(* Logix 5000 AddOnInstructionDefinition export Banner_K50Z_Param_v4; software revision 33.00; part 2 of 3 *)
(* tags used below, declared in another part *)
   K50Z : Banner_K50Z_v4;
   Port_Data : Banner_IOL_Port_v4;
   Port : DINT;
   Local_Control : DINT;
   Command_Being_Processed : BOOL;
   Update_Archive : BOOL;
   Index_Write_Inprocess : INT;
   Index_Write_Control : INT;
   Inprocess_Index : DINT;
(* Banner_K50Z_Param_v4, continued *)

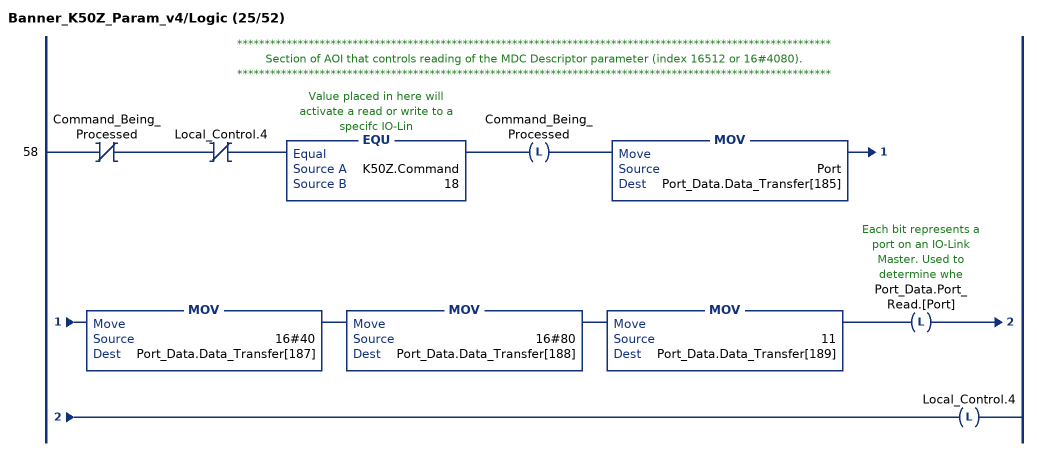
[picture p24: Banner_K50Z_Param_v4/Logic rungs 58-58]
   // ************************************************************************************************************
   // Section of AOI that controls reading of the MDC Descriptor parameter (index 16512 or 16#4080).
   // ************************************************************************************************************
   58: XIO(Command_Being_Processed)XIO(Local_Control.4)EQU(K50Z.Command,18)OTL(Command_Being_Processed)MOV(Port,Port_Data.Data_Transfer[185])MOV(16#40,Port_Data.Data_Transfer[187])MOV(16#80,Port_Data.Data_Transfer[188])MOV(11,Port_Data.Data_Transfer[189])OTL(Port_Data.Port_Read.[Port])OTL(Local_Control.4);
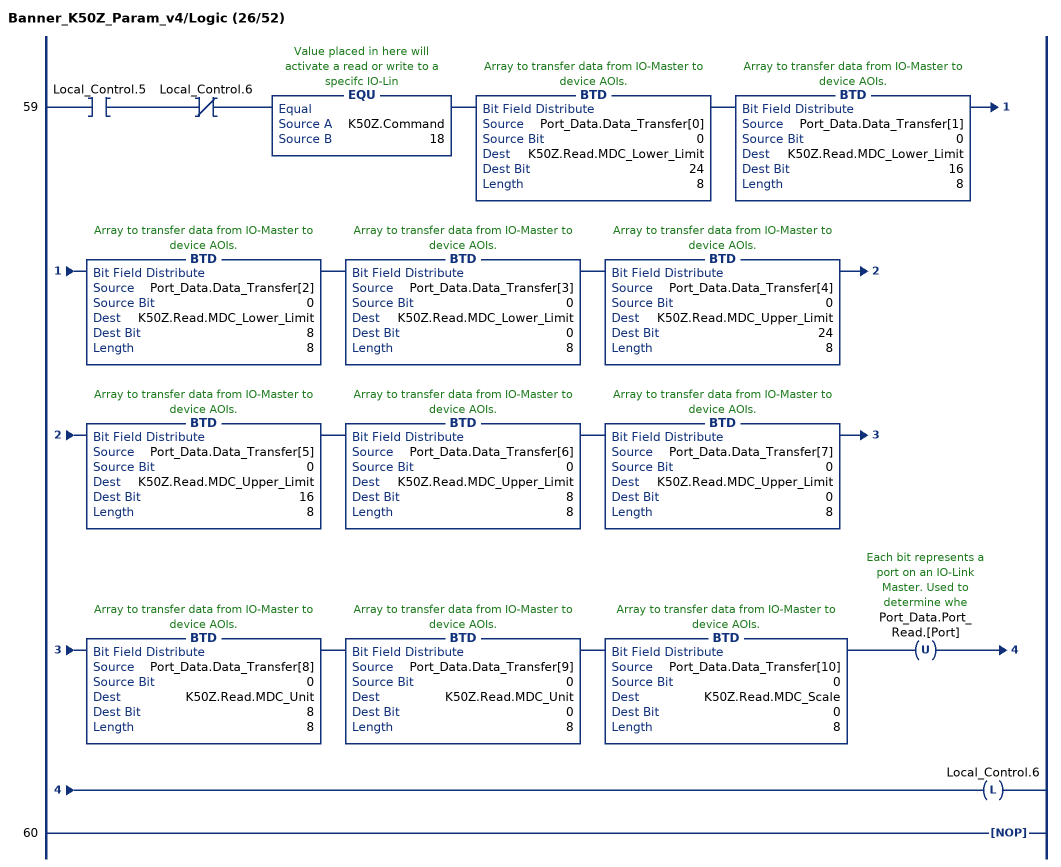
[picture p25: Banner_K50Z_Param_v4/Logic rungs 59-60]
   59: XIC(Local_Control.5)XIO(Local_Control.6)EQU(K50Z.Command,18)BTD(Port_Data.Data_Transfer[0],0,K50Z.Read.MDC_Lower_Limit,24,8)BTD(Port_Data.Data_Transfer[1],0,K50Z.Read.MDC_Lower_Limit,16,8)BTD(Port_Data.Data_Transfer[2],0,K50Z.Read.MDC_Lower_Limit,8,8)BTD(Port_Data.Data_Transfer[3],0,K50Z.Read.MDC_Lower_Limit,0,8)BTD(Port_Data.Data_Transfer[4],0,K50Z.Read.MDC_Upper_Limit,24,8)BTD(Port_Data.Data_Transfer[5],0,K50Z.Read.MDC_Upper_Limit,16,8)BTD(Port_Data.Data_Transfer[6],0,K50Z.Read.MDC_Upper_Limit,8,8)BTD(Port_Data.Data_Transfer[7],0,K50Z.Read.MDC_Upper_Limit,0,8)BTD(Port_Data.Data_Transfer[8],0,K50Z.Read.MDC_Unit,8,8)BTD(Port_Data.Data_Transfer[9],0,K50Z.Read.MDC_Unit,0,8)BTD(Port_Data.Data_Transfer[10],0,K50Z.Read.MDC_Scale,0,8)OTU(Port_Data.Port_Read.[Port])OTL(Local_Control.6);
   60: NOP();
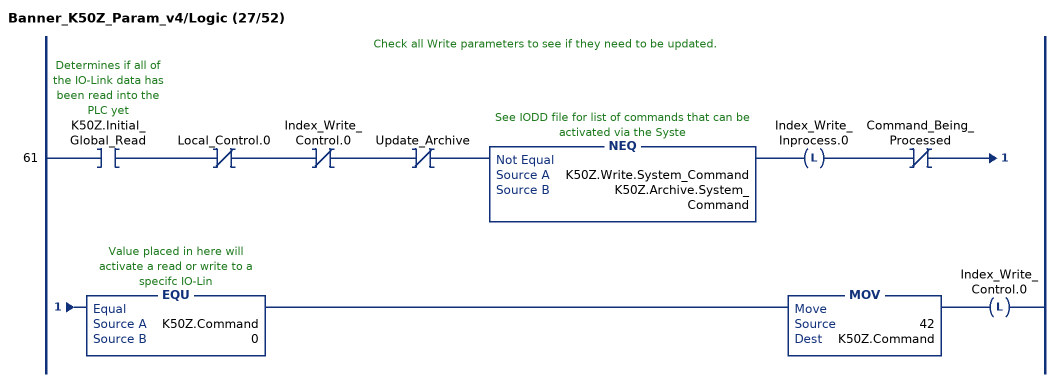
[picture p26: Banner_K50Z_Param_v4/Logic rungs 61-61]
   // Check all Write parameters to see if they need to be updated.
   61: XIC(K50Z.Initial_Global_Read)XIO(Local_Control.0)XIO(Index_Write_Control.0)XIO(Update_Archive)NEQ(K50Z.Write.System_Command,K50Z.Archive.System_Command)OTL(Index_Write_Inprocess.0)XIO(Command_Being_Processed)EQU(K50Z.Command,0)MOV(42,K50Z.Command)OTL(Index_Write_Control.0);
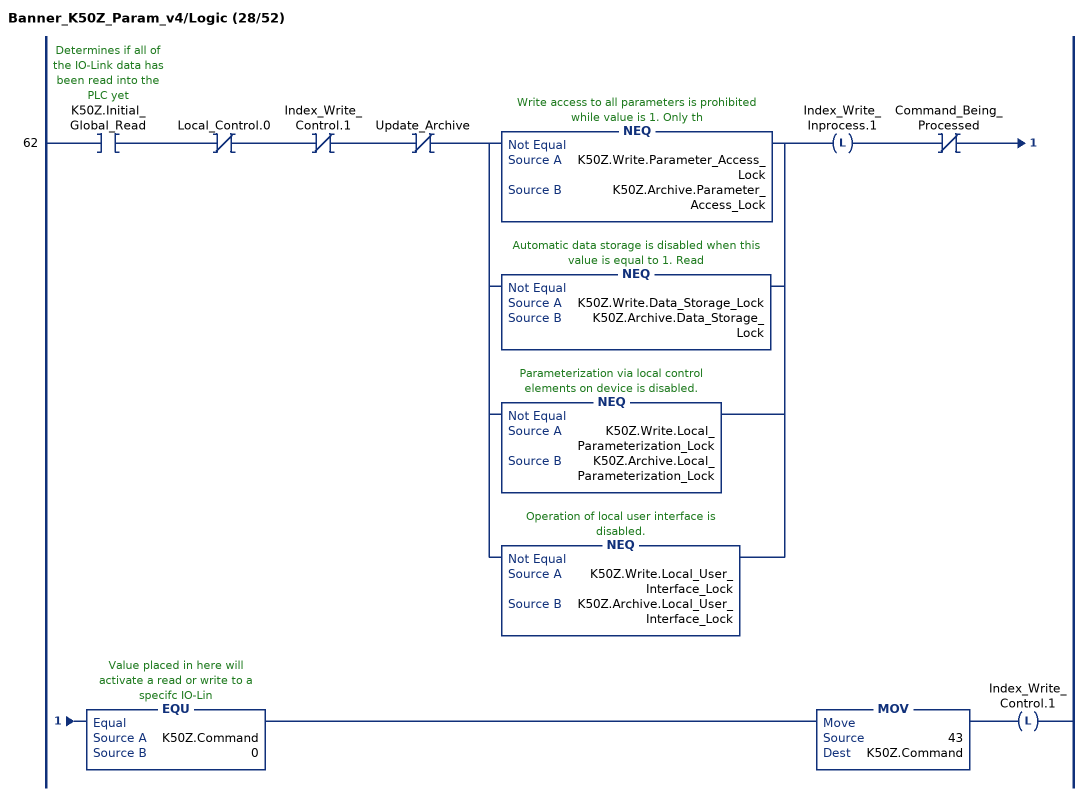
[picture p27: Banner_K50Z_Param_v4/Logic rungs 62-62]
   62: XIC(K50Z.Initial_Global_Read)XIO(Local_Control.0)XIO(Index_Write_Control.1)XIO(Update_Archive)[NEQ(K50Z.Write.Parameter_Access_Lock,K50Z.Archive.Parameter_Access_Lock) ,NEQ(K50Z.Write.Data_Storage_Lock,K50Z.Archive.Data_Storage_Lock) ,NEQ(K50Z.Write.Local_Parameterization_Lock,K50Z.Archive.Local_Parameterization_Lock) ,NEQ(K50Z.Write.Local_User_Interface_Lock,K50Z.Archive.Local_User_Interface_Lock) ]OTL(Index_Write_Inprocess.1)XIO(Command_Being_Processed)EQU(K50Z.Command,0)MOV(43,K50Z.Command)OTL(Index_Write_Control.1);
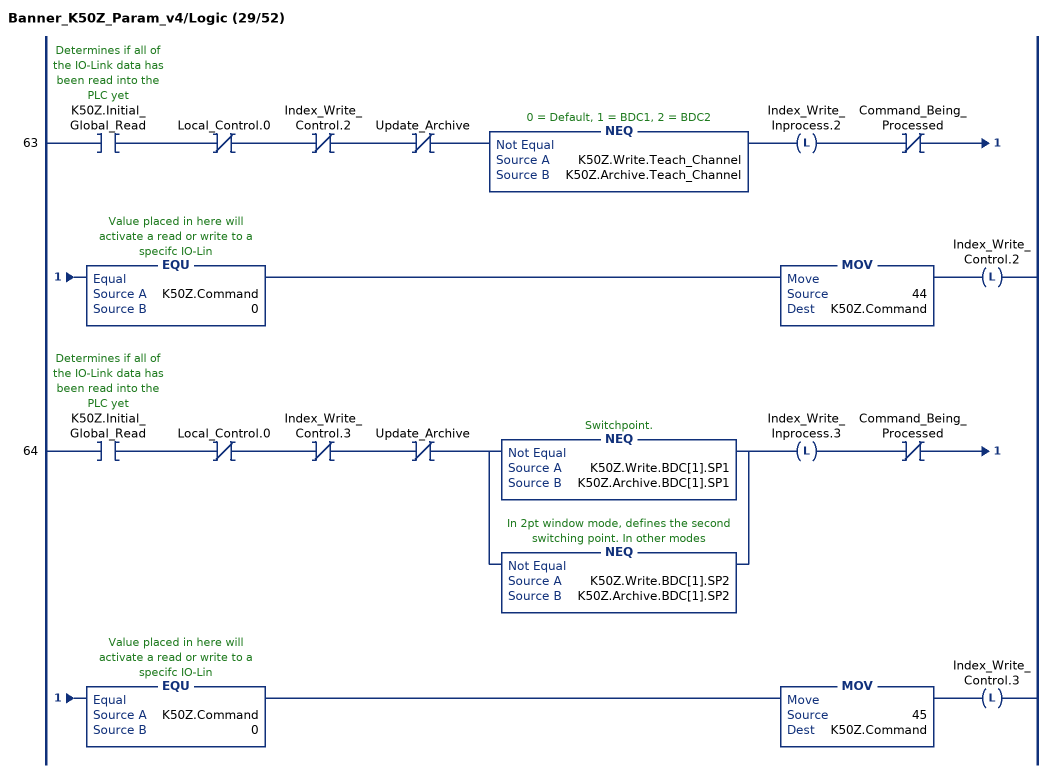
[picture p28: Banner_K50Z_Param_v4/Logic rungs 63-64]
   63: XIC(K50Z.Initial_Global_Read)XIO(Local_Control.0)XIO(Index_Write_Control.2)XIO(Update_Archive)NEQ(K50Z.Write.Teach_Channel,K50Z.Archive.Teach_Channel)OTL(Index_Write_Inprocess.2)XIO(Command_Being_Processed)EQU(K50Z.Command,0)MOV(44,K50Z.Command)OTL(Index_Write_Control.2);
   64: XIC(K50Z.Initial_Global_Read)XIO(Local_Control.0)XIO(Index_Write_Control.3)XIO(Update_Archive)[NEQ(K50Z.Write.BDC[1].SP1,K50Z.Archive.BDC[1].SP1) ,NEQ(K50Z.Write.BDC[1].SP2,K50Z.Archive.BDC[1].SP2) ]OTL(Index_Write_Inprocess.3)XIO(Command_Being_Processed)EQU(K50Z.Command,0)MOV(45,K50Z.Command)OTL(Index_Write_Control.3);
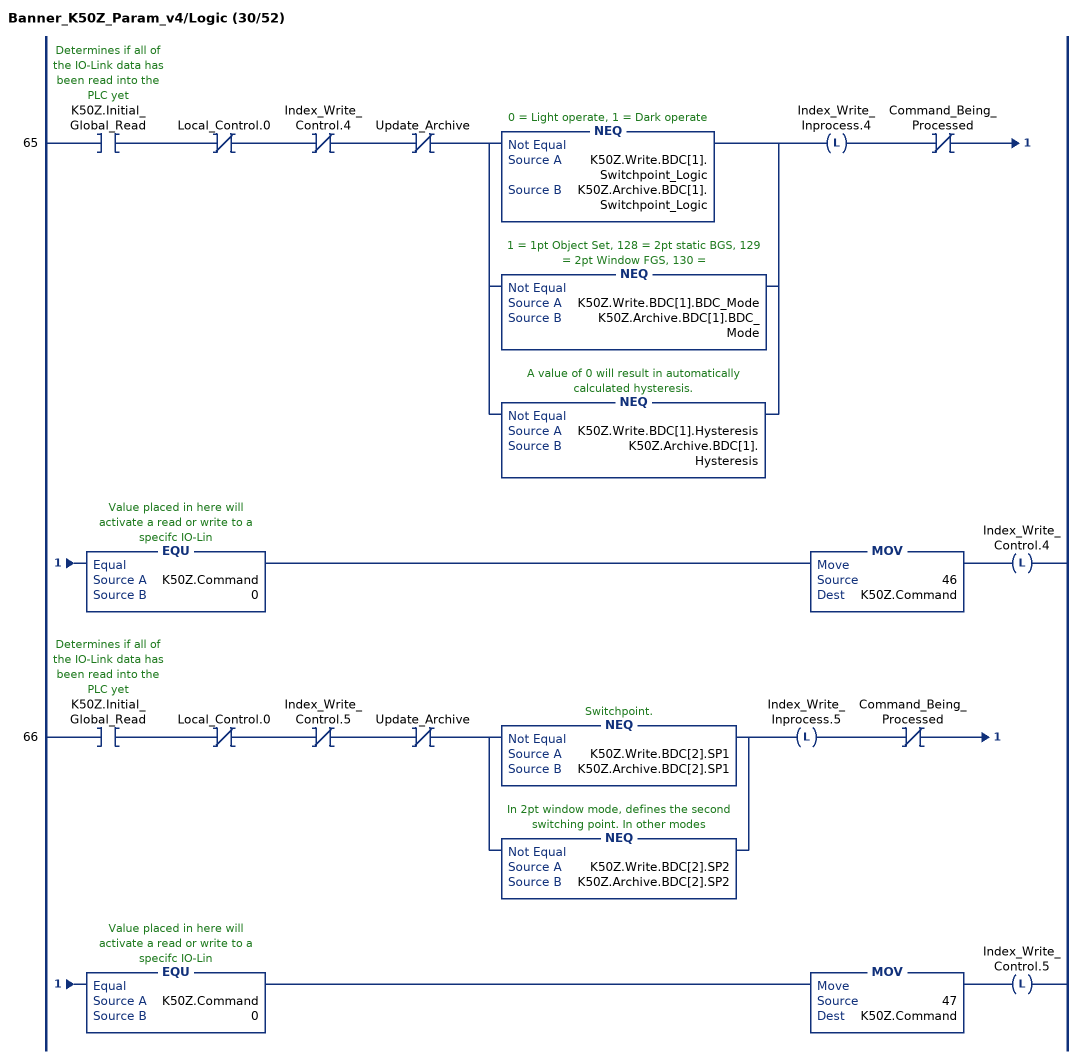
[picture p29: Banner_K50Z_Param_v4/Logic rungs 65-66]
   65: XIC(K50Z.Initial_Global_Read)XIO(Local_Control.0)XIO(Index_Write_Control.4)XIO(Update_Archive)[NEQ(K50Z.Write.BDC[1].Switchpoint_Logic,K50Z.Archive.BDC[1].Switchpoint_Logic) ,NEQ(K50Z.Write.BDC[1].BDC_Mode,K50Z.Archive.BDC[1].BDC_Mode) ,NEQ(K50Z.Write.BDC[1].Hysteresis,K50Z.Archive.BDC[1].Hysteresis) ]OTL(Index_Write_Inprocess.4)XIO(Command_Being_Processed)EQU(K50Z.Command,0)MOV(46,K50Z.Command)OTL(Index_Write_Control.4);
   66: XIC(K50Z.Initial_Global_Read)XIO(Local_Control.0)XIO(Index_Write_Control.5)XIO(Update_Archive)[NEQ(K50Z.Write.BDC[2].SP1,K50Z.Archive.BDC[2].SP1) ,NEQ(K50Z.Write.BDC[2].SP2,K50Z.Archive.BDC[2].SP2) ]OTL(Index_Write_Inprocess.5)XIO(Command_Being_Processed)EQU(K50Z.Command,0)MOV(47,K50Z.Command)OTL(Index_Write_Control.5);
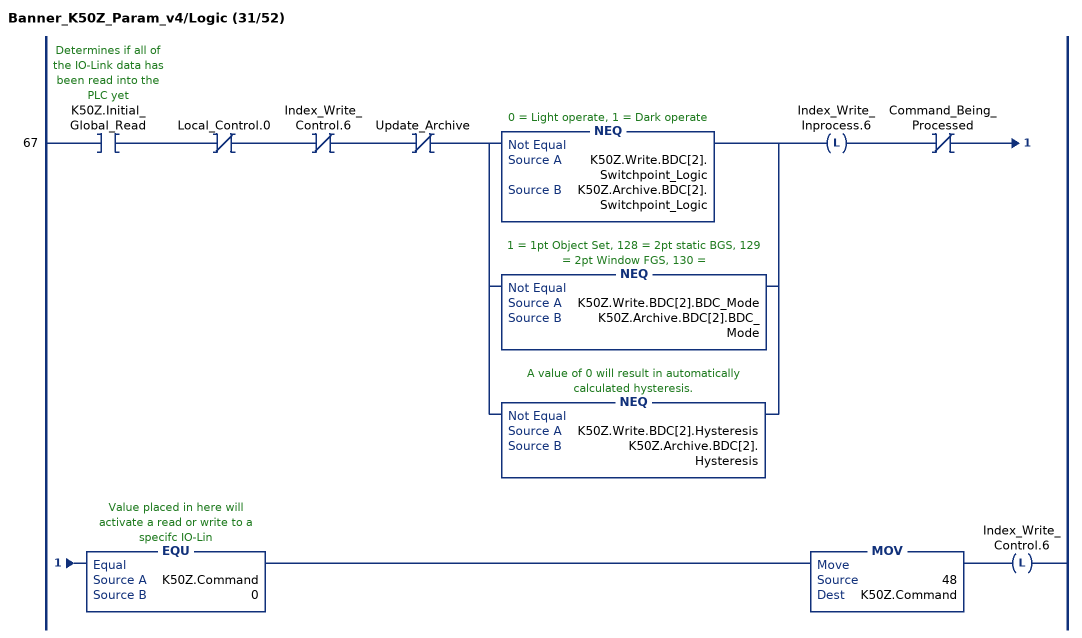
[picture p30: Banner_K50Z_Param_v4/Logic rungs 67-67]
   67: XIC(K50Z.Initial_Global_Read)XIO(Local_Control.0)XIO(Index_Write_Control.6)XIO(Update_Archive)[NEQ(K50Z.Write.BDC[2].Switchpoint_Logic,K50Z.Archive.BDC[2].Switchpoint_Logic) ,NEQ(K50Z.Write.BDC[2].BDC_Mode,K50Z.Archive.BDC[2].BDC_Mode) ,NEQ(K50Z.Write.BDC[2].Hysteresis,K50Z.Archive.BDC[2].Hysteresis) ]OTL(Index_Write_Inprocess.6)XIO(Command_Being_Processed)EQU(K50Z.Command,0)MOV(48,K50Z.Command)OTL(Index_Write_Control.6);
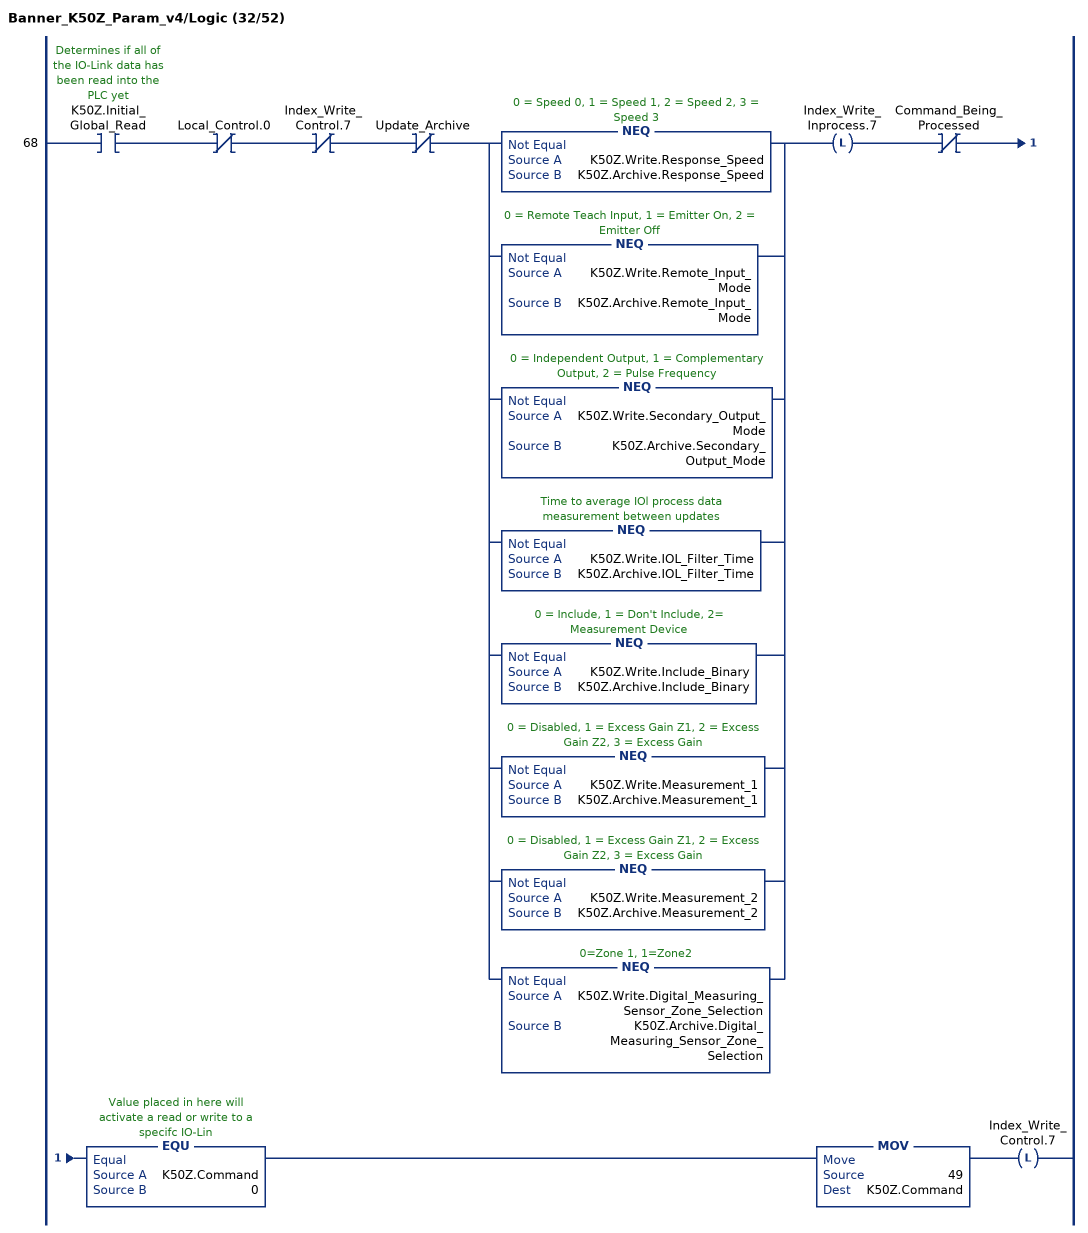
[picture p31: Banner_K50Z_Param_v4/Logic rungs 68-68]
   68: XIC(K50Z.Initial_Global_Read)XIO(Local_Control.0)XIO(Index_Write_Control.7)XIO(Update_Archive)[NEQ(K50Z.Write.Response_Speed,K50Z.Archive.Response_Speed) ,NEQ(K50Z.Write.Remote_Input_Mode,K50Z.Archive.Remote_Input_Mode) ,NEQ(K50Z.Write.Secondary_Output_Mode,K50Z.Archive.Secondary_Output_Mode) ,NEQ(K50Z.Write.IOL_Filter_Time,K50Z.Archive.IOL_Filter_Time) ,NEQ(K50Z.Write.Include_Binary,K50Z.Archive.Include_Binary) ,NEQ(K50Z.Write.Measurement_1,K50Z.Archive.Measurement_1) ,NEQ(K50Z.Write.Measurement_2,K50Z.Archive.Measurement_2) ,NEQ(K50Z.Write.Digital_Measuring_Sensor_Zone_Selection,K50Z.Archive.Digital_Measuring_Sensor_Zone_Selection) ]OTL(Index_Write_Inprocess.7)XIO(Command_Being_Processed)EQU(K50Z.Command,0)MOV(49,K50Z.Command)OTL(Index_Write_Control.7);
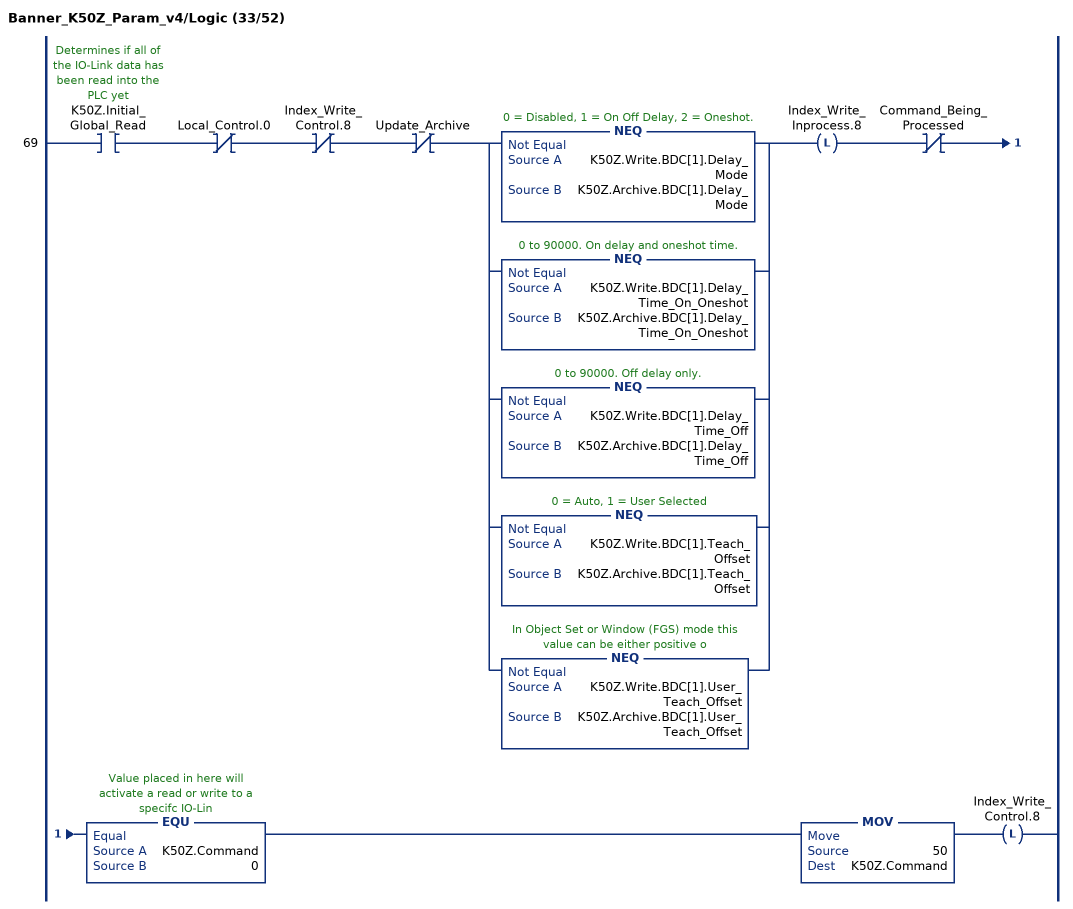
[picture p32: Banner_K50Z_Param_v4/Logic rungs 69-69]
   69: XIC(K50Z.Initial_Global_Read)XIO(Local_Control.0)XIO(Index_Write_Control.8)XIO(Update_Archive)[NEQ(K50Z.Write.BDC[1].Delay_Mode,K50Z.Archive.BDC[1].Delay_Mode) ,NEQ(K50Z.Write.BDC[1].Delay_Time_On_Oneshot,K50Z.Archive.BDC[1].Delay_Time_On_Oneshot) ,NEQ(K50Z.Write.BDC[1].Delay_Time_Off,K50Z.Archive.BDC[1].Delay_Time_Off) ,NEQ(K50Z.Write.BDC[1].Teach_Offset,K50Z.Archive.BDC[1].Teach_Offset) ,NEQ(K50Z.Write.BDC[1].User_Teach_Offset,K50Z.Archive.BDC[1].User_Teach_Offset) ]OTL(Index_Write_Inprocess.8)XIO(Command_Being_Processed)EQU(K50Z.Command,0)MOV(50,K50Z.Command)OTL(Index_Write_Control.8);
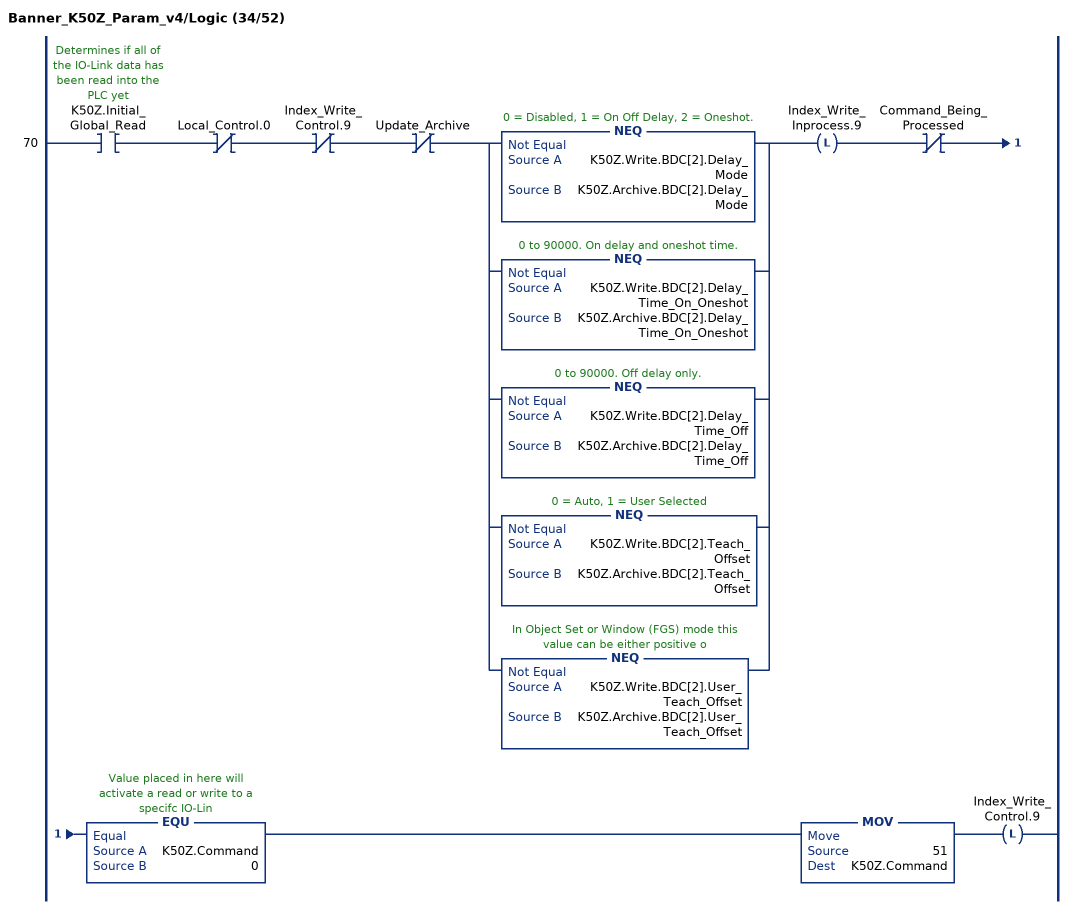
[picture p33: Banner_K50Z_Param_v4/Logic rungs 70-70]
   70: XIC(K50Z.Initial_Global_Read)XIO(Local_Control.0)XIO(Index_Write_Control.9)XIO(Update_Archive)[NEQ(K50Z.Write.BDC[2].Delay_Mode,K50Z.Archive.BDC[2].Delay_Mode) ,NEQ(K50Z.Write.BDC[2].Delay_Time_On_Oneshot,K50Z.Archive.BDC[2].Delay_Time_On_Oneshot) ,NEQ(K50Z.Write.BDC[2].Delay_Time_Off,K50Z.Archive.BDC[2].Delay_Time_Off) ,NEQ(K50Z.Write.BDC[2].Teach_Offset,K50Z.Archive.BDC[2].Teach_Offset) ,NEQ(K50Z.Write.BDC[2].User_Teach_Offset,K50Z.Archive.BDC[2].User_Teach_Offset) ]OTL(Index_Write_Inprocess.9)XIO(Command_Being_Processed)EQU(K50Z.Command,0)MOV(51,K50Z.Command)OTL(Index_Write_Control.9);
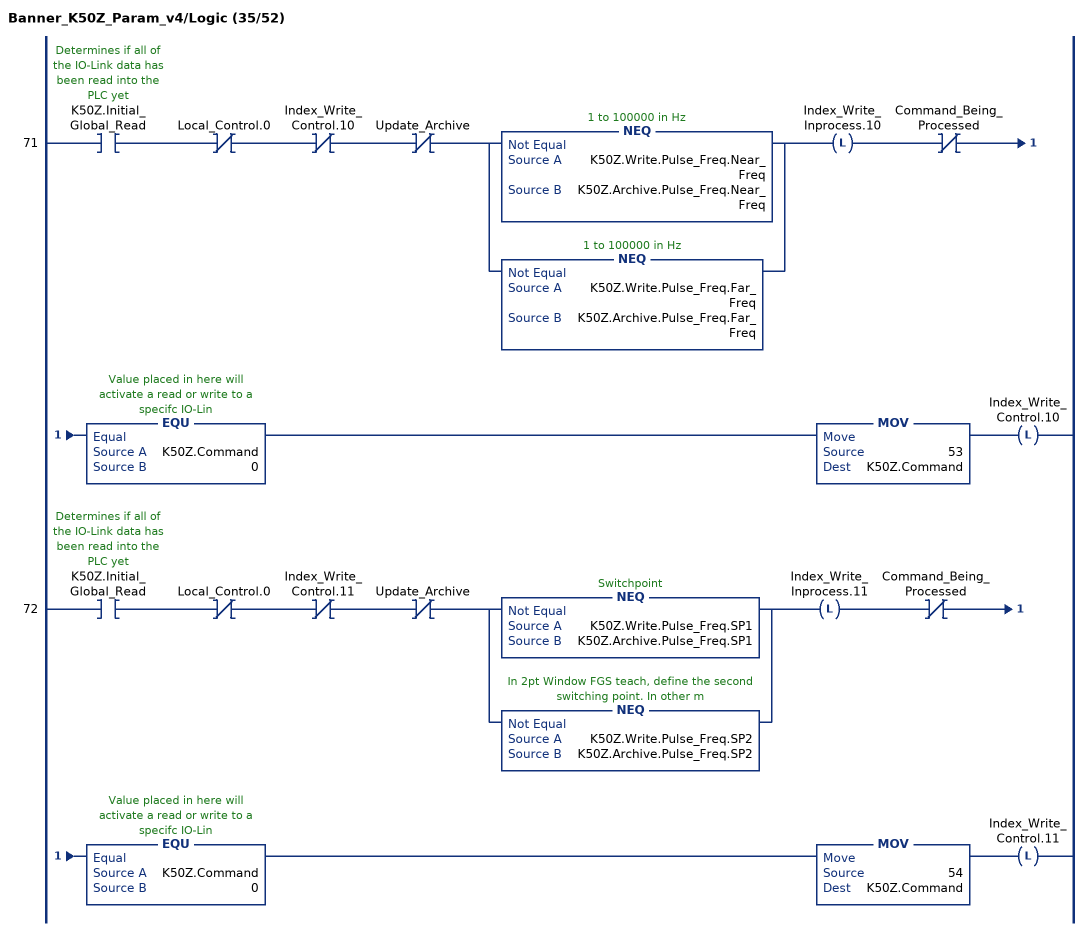
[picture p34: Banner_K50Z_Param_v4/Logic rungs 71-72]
   71: XIC(K50Z.Initial_Global_Read)XIO(Local_Control.0)XIO(Index_Write_Control.10)XIO(Update_Archive)[NEQ(K50Z.Write.Pulse_Freq.Near_Freq,K50Z.Archive.Pulse_Freq.Near_Freq) ,NEQ(K50Z.Write.Pulse_Freq.Far_Freq,K50Z.Archive.Pulse_Freq.Far_Freq) ]OTL(Index_Write_Inprocess.10)XIO(Command_Being_Processed)EQU(K50Z.Command,0)MOV(53,K50Z.Command)OTL(Index_Write_Control.10);
   72: XIC(K50Z.Initial_Global_Read)XIO(Local_Control.0)XIO(Index_Write_Control.11)XIO(Update_Archive)[NEQ(K50Z.Write.Pulse_Freq.SP1,K50Z.Archive.Pulse_Freq.SP1) ,NEQ(K50Z.Write.Pulse_Freq.SP2,K50Z.Archive.Pulse_Freq.SP2) ]OTL(Index_Write_Inprocess.11)XIO(Command_Being_Processed)EQU(K50Z.Command,0)MOV(54,K50Z.Command)OTL(Index_Write_Control.11);
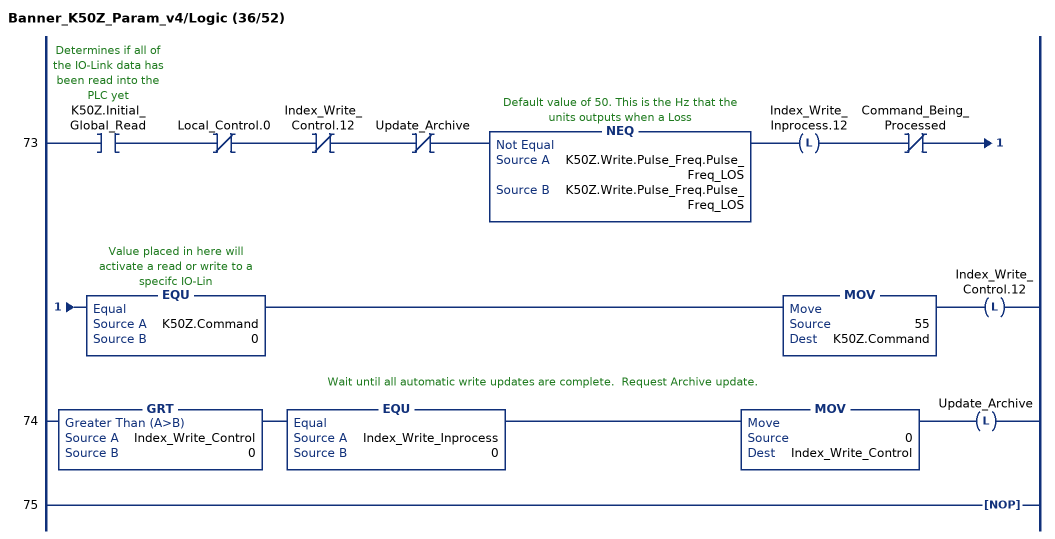
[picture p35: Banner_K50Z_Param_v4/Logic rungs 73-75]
   73: XIC(K50Z.Initial_Global_Read)XIO(Local_Control.0)XIO(Index_Write_Control.12)XIO(Update_Archive)NEQ(K50Z.Write.Pulse_Freq.Pulse_Freq_LOS,K50Z.Write.Pulse_Freq.Pulse_Freq_LOS)OTL(Index_Write_Inprocess.12)XIO(Command_Being_Processed)EQU(K50Z.Command,0)MOV(55,K50Z.Command)OTL(Index_Write_Control.12);
   // Wait until all automatic write updates are complete.  Request Archive update.
   74: GRT(Index_Write_Control,0)EQU(Index_Write_Inprocess,0)MOV(0,Index_Write_Control)OTL(Update_Archive);
   75: NOP();
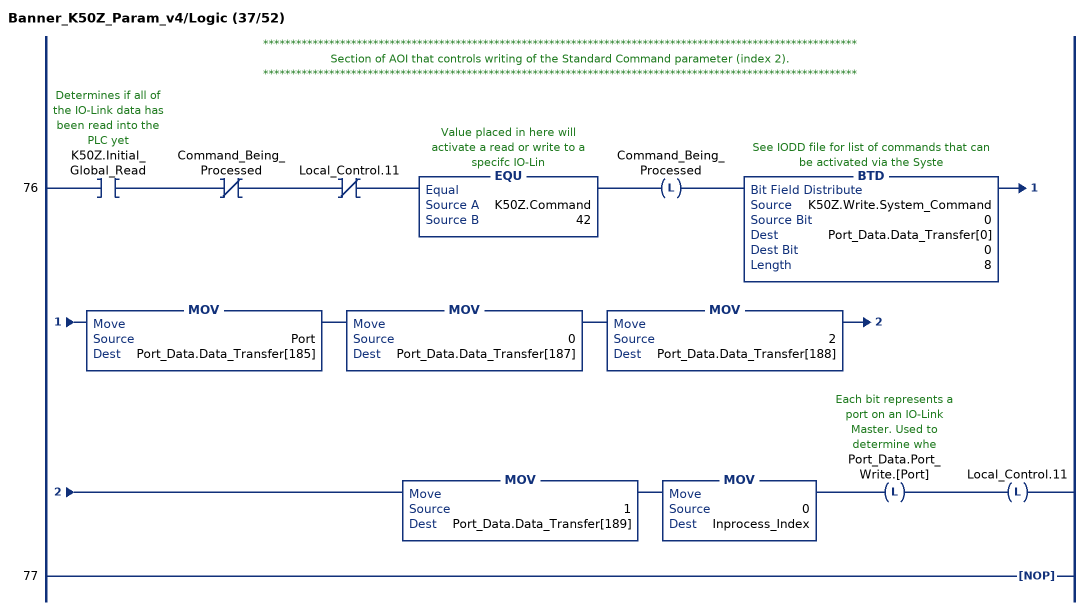
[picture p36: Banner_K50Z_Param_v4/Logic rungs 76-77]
   // ************************************************************************************************************
   // Section of AOI that controls writing of the Standard Command parameter (index 2).
   // ************************************************************************************************************
   76: XIC(K50Z.Initial_Global_Read)XIO(Command_Being_Processed)XIO(Local_Control.11)EQU(K50Z.Command,42)OTL(Command_Being_Processed)BTD(K50Z.Write.System_Command,0,Port_Data.Data_Transfer[0],0,8)MOV(Port,Port_Data.Data_Transfer[185])MOV(0,Port_Data.Data_Transfer[187])MOV(2,Port_Data.Data_Transfer[188])MOV(1,Port_Data.Data_Transfer[189])MOV(0,Inprocess_Index)OTL(Port_Data.Port_Write.[Port])OTL(Local_Control.11);
   77: NOP();
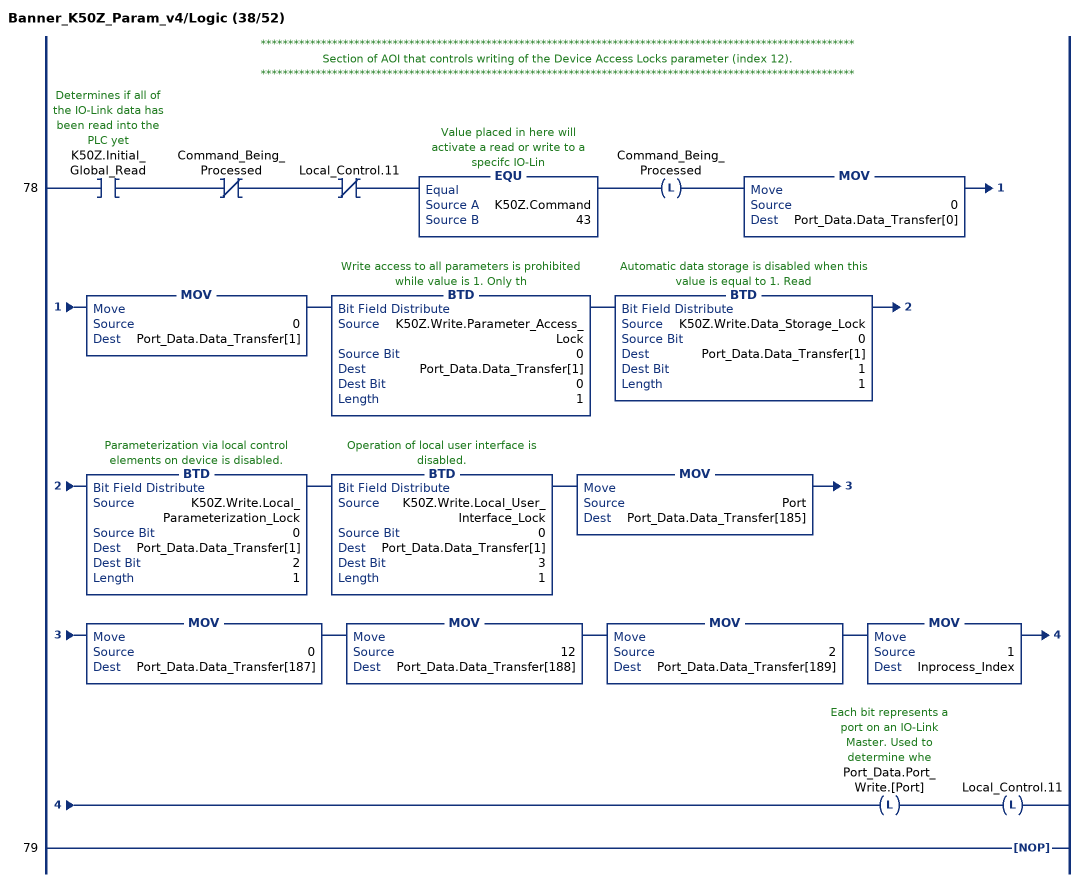
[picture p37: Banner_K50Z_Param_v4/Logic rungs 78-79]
   // ************************************************************************************************************
   // Section of AOI that controls writing of the Device Access Locks parameter (index 12).
   // ************************************************************************************************************
   78: XIC(K50Z.Initial_Global_Read)XIO(Command_Being_Processed)XIO(Local_Control.11)EQU(K50Z.Command,43)OTL(Command_Being_Processed)MOV(0,Port_Data.Data_Transfer[0])MOV(0,Port_Data.Data_Transfer[1])BTD(K50Z.Write.Parameter_Access_Lock,0,Port_Data.Data_Transfer[1],0,1)BTD(K50Z.Write.Data_Storage_Lock,0,Port_Data.Data_Transfer[1],1,1)BTD(K50Z.Write.Local_Parameterization_Lock,0,Port_Data.Data_Transfer[1],2,1)BTD(K50Z.Write.Local_User_Interface_Lock,0,Port_Data.Data_Transfer[1],3,1)MOV(Port,Port_Data.Data_Transfer[185])MOV(0,Port_Data.Data_Transfer[187])MOV(12,Port_Data.Data_Transfer[188])MOV(2,Port_Data.Data_Transfer[189])MOV(1,Inprocess_Index)OTL(Port_Data.Port_Write.[Port])OTL(Local_Control.11);
   79: NOP();
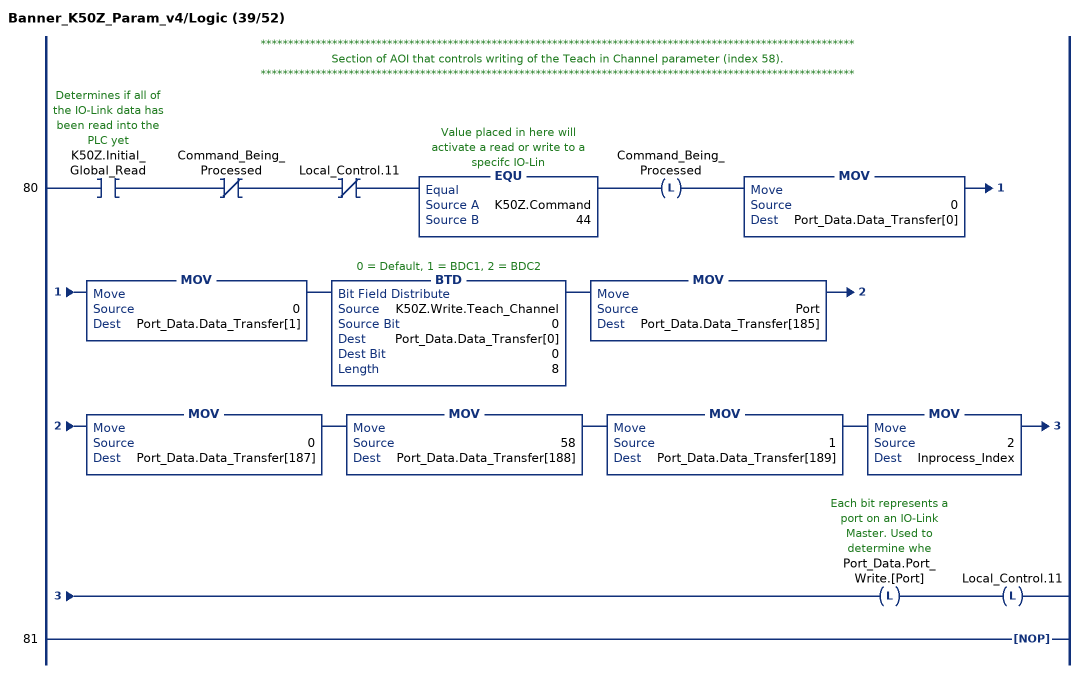
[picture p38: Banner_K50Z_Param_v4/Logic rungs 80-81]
   // ************************************************************************************************************
   // Section of AOI that controls writing of the Teach in Channel parameter (index 58).
   // ************************************************************************************************************
   80: XIC(K50Z.Initial_Global_Read)XIO(Command_Being_Processed)XIO(Local_Control.11)EQU(K50Z.Command,44)OTL(Command_Being_Processed)MOV(0,Port_Data.Data_Transfer[0])MOV(0,Port_Data.Data_Transfer[1])BTD(K50Z.Write.Teach_Channel,0,Port_Data.Data_Transfer[0],0,8)MOV(Port,Port_Data.Data_Transfer[185])MOV(0,Port_Data.Data_Transfer[187])MOV(58,Port_Data.Data_Transfer[188])MOV(1,Port_Data.Data_Transfer[189])MOV(2,Inprocess_Index)OTL(Port_Data.Port_Write.[Port])OTL(Local_Control.11);
   81: NOP();
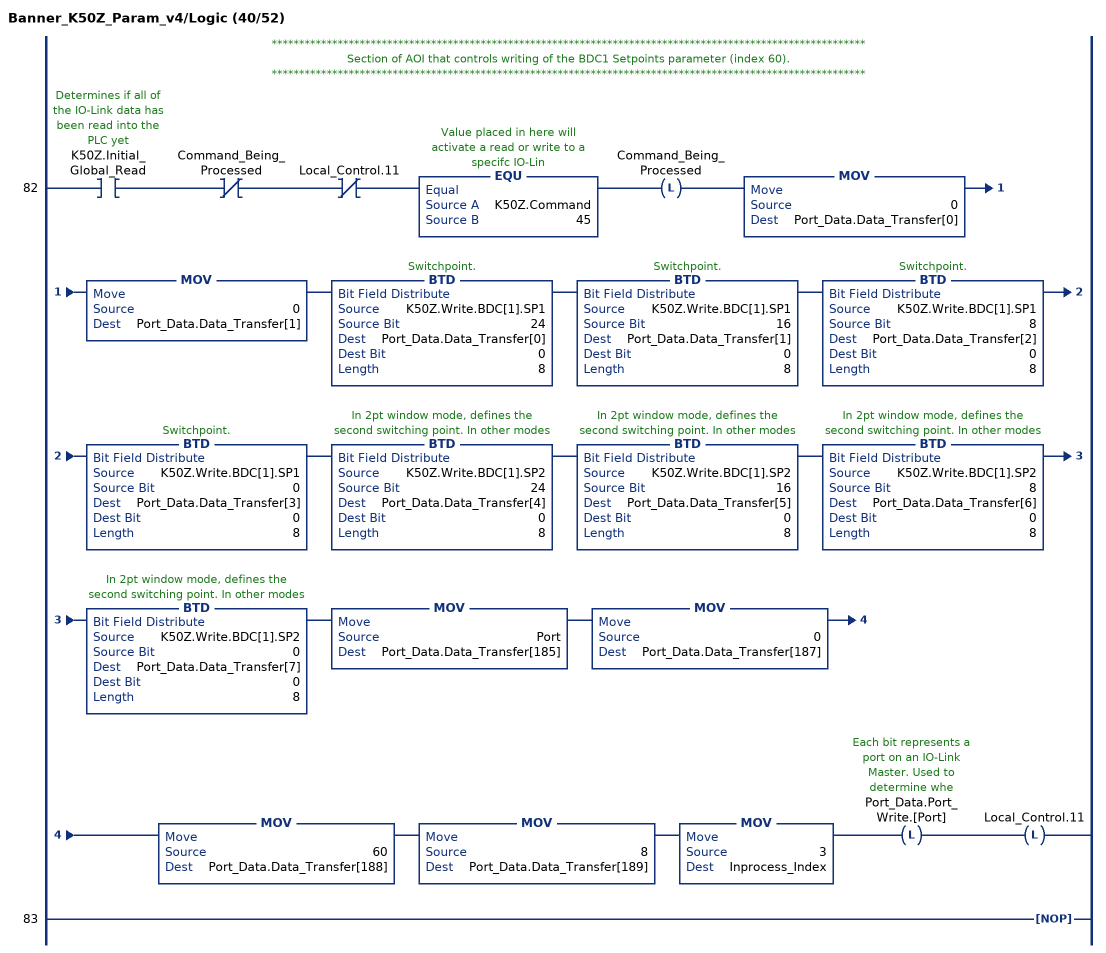
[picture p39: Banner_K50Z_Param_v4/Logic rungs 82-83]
   // ************************************************************************************************************
   // Section of AOI that controls writing of the BDC1 Setpoints parameter (index 60).
   // ************************************************************************************************************
   82: XIC(K50Z.Initial_Global_Read)XIO(Command_Being_Processed)XIO(Local_Control.11)EQU(K50Z.Command,45)OTL(Command_Being_Processed)MOV(0,Port_Data.Data_Transfer[0])MOV(0,Port_Data.Data_Transfer[1])BTD(K50Z.Write.BDC[1].SP1,24,Port_Data.Data_Transfer[0],0,8)BTD(K50Z.Write.BDC[1].SP1,16,Port_Data.Data_Transfer[1],0,8)BTD(K50Z.Write.BDC[1].SP1,8,Port_Data.Data_Transfer[2],0,8)BTD(K50Z.Write.BDC[1].SP1,0,Port_Data.Data_Transfer[3],0,8)BTD(K50Z.Write.BDC[1].SP2,24,Port_Data.Data_Transfer[4],0,8)BTD(K50Z.Write.BDC[1].SP2,16,Port_Data.Data_Transfer[5],0,8)BTD(K50Z.Write.BDC[1].SP2,8,Port_Data.Data_Transfer[6],0,8)BTD(K50Z.Write.BDC[1].SP2,0,Port_Data.Data_Transfer[7],0,8)MOV(Port,Port_Data.Data_Transfer[185])MOV(0,Port_Data.Data_Transfer[187])MOV(60,Port_Data.Data_Transfer[188])MOV(8,Port_Data.Data_Transfer[189])MOV(3,Inprocess_Index)OTL(Port_Data.Port_Write.[Port])OTL(Local_Control.11);
   83: NOP();
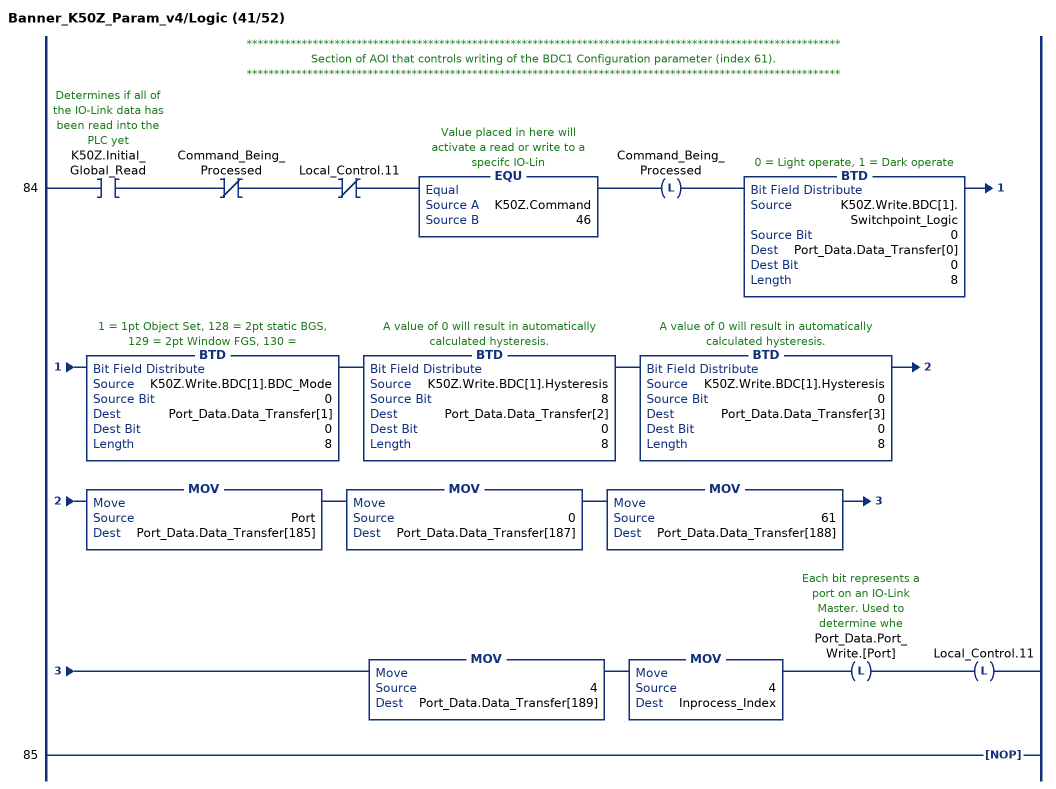
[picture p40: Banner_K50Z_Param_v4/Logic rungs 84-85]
   // ************************************************************************************************************
   // Section of AOI that controls writing of the BDC1 Configuration parameter (index 61).
   // ************************************************************************************************************
   84: XIC(K50Z.Initial_Global_Read)XIO(Command_Being_Processed)XIO(Local_Control.11)EQU(K50Z.Command,46)OTL(Command_Being_Processed)BTD(K50Z.Write.BDC[1].Switchpoint_Logic,0,Port_Data.Data_Transfer[0],0,8)BTD(K50Z.Write.BDC[1].BDC_Mode,0,Port_Data.Data_Transfer[1],0,8)BTD(K50Z.Write.BDC[1].Hysteresis,8,Port_Data.Data_Transfer[2],0,8)BTD(K50Z.Write.BDC[1].Hysteresis,0,Port_Data.Data_Transfer[3],0,8)MOV(Port,Port_Data.Data_Transfer[185])MOV(0,Port_Data.Data_Transfer[187])MOV(61,Port_Data.Data_Transfer[188])MOV(4,Port_Data.Data_Transfer[189])MOV(4,Inprocess_Index)OTL(Port_Data.Port_Write.[Port])OTL(Local_Control.11);
   85: NOP();
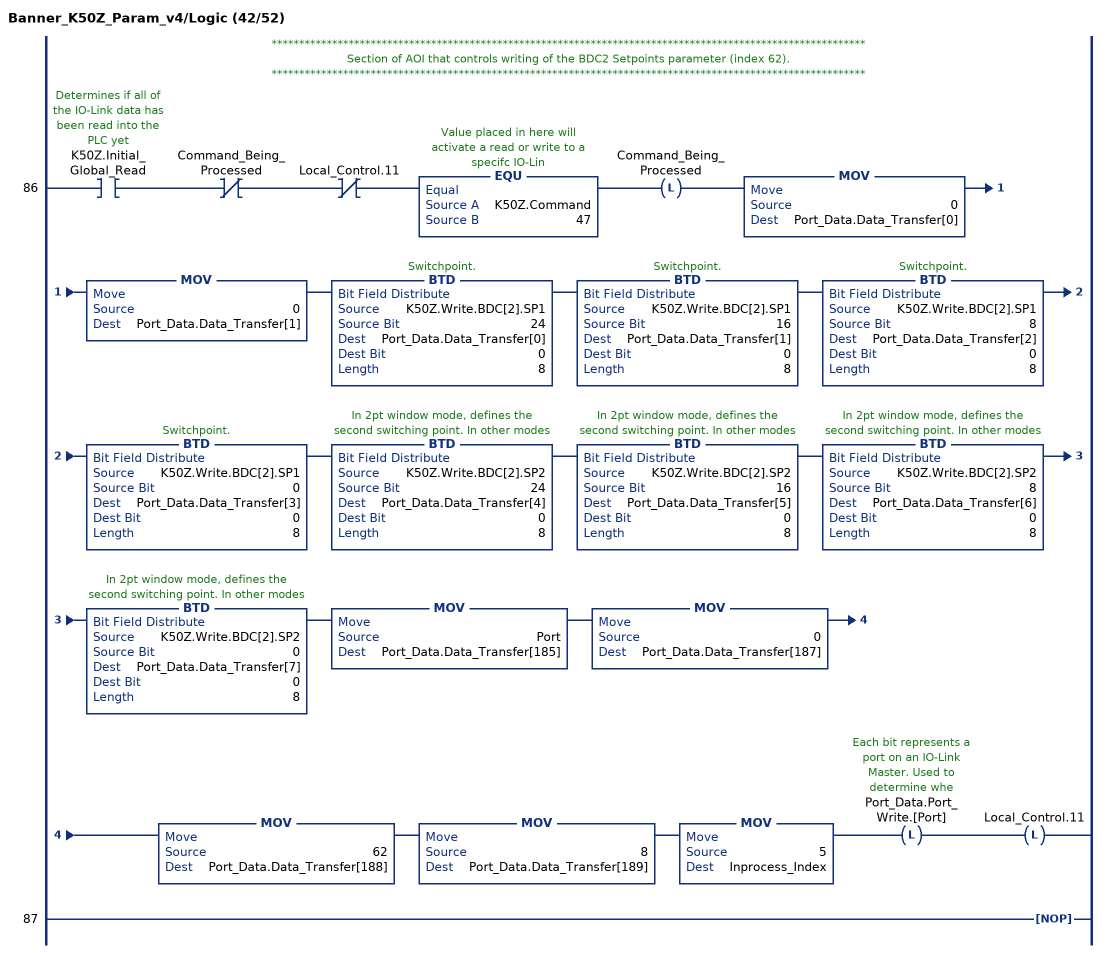
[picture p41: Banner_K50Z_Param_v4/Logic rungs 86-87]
   // ************************************************************************************************************
   // Section of AOI that controls writing of the BDC2 Setpoints parameter (index 62).
   // ************************************************************************************************************
   86: XIC(K50Z.Initial_Global_Read)XIO(Command_Being_Processed)XIO(Local_Control.11)EQU(K50Z.Command,47)OTL(Command_Being_Processed)MOV(0,Port_Data.Data_Transfer[0])MOV(0,Port_Data.Data_Transfer[1])BTD(K50Z.Write.BDC[2].SP1,24,Port_Data.Data_Transfer[0],0,8)BTD(K50Z.Write.BDC[2].SP1,16,Port_Data.Data_Transfer[1],0,8)BTD(K50Z.Write.BDC[2].SP1,8,Port_Data.Data_Transfer[2],0,8)BTD(K50Z.Write.BDC[2].SP1,0,Port_Data.Data_Transfer[3],0,8)BTD(K50Z.Write.BDC[2].SP2,24,Port_Data.Data_Transfer[4],0,8)BTD(K50Z.Write.BDC[2].SP2,16,Port_Data.Data_Transfer[5],0,8)BTD(K50Z.Write.BDC[2].SP2,8,Port_Data.Data_Transfer[6],0,8)BTD(K50Z.Write.BDC[2].SP2,0,Port_Data.Data_Transfer[7],0,8)MOV(Port,Port_Data.Data_Transfer[185])MOV(0,Port_Data.Data_Transfer[187])MOV(62,Port_Data.Data_Transfer[188])MOV(8,Port_Data.Data_Transfer[189])MOV(5,Inprocess_Index)OTL(Port_Data.Port_Write.[Port])OTL(Local_Control.11);
   87: NOP();
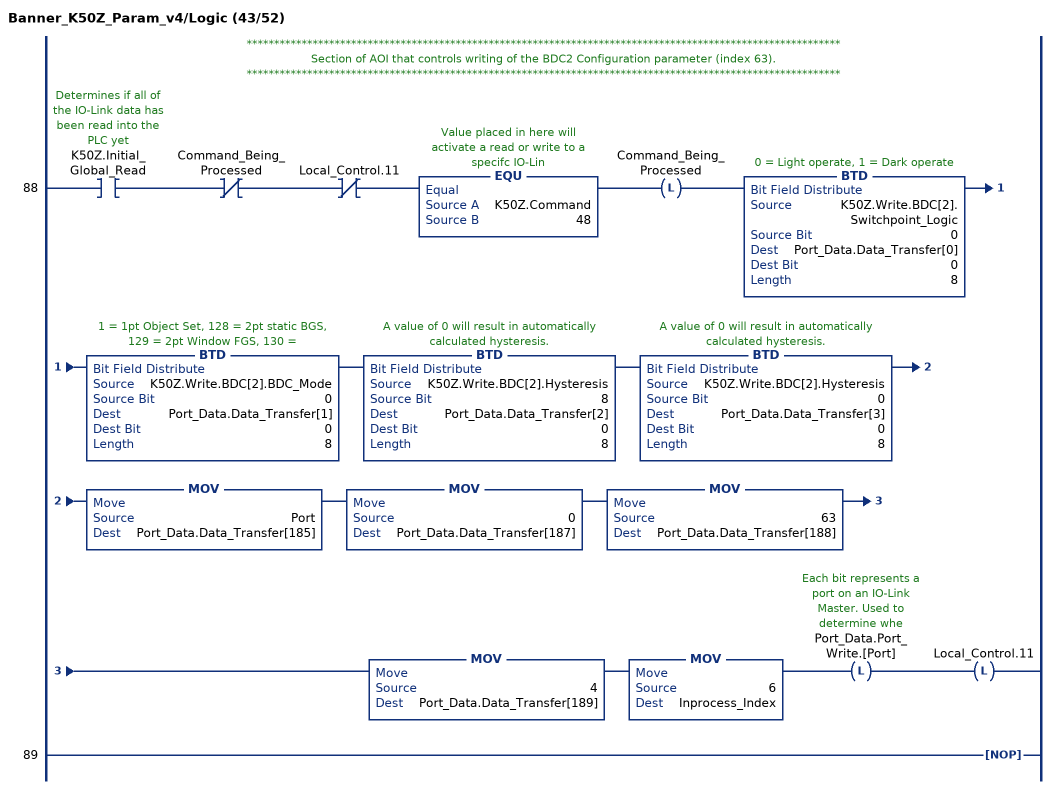
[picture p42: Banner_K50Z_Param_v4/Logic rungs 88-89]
   // ************************************************************************************************************
   // Section of AOI that controls writing of the BDC2 Configuration parameter (index 63).
   // ************************************************************************************************************
   88: XIC(K50Z.Initial_Global_Read)XIO(Command_Being_Processed)XIO(Local_Control.11)EQU(K50Z.Command,48)OTL(Command_Being_Processed)BTD(K50Z.Write.BDC[2].Switchpoint_Logic,0,Port_Data.Data_Transfer[0],0,8)BTD(K50Z.Write.BDC[2].BDC_Mode,0,Port_Data.Data_Transfer[1],0,8)BTD(K50Z.Write.BDC[2].Hysteresis,8,Port_Data.Data_Transfer[2],0,8)BTD(K50Z.Write.BDC[2].Hysteresis,0,Port_Data.Data_Transfer[3],0,8)MOV(Port,Port_Data.Data_Transfer[185])MOV(0,Port_Data.Data_Transfer[187])MOV(63,Port_Data.Data_Transfer[188])MOV(4,Port_Data.Data_Transfer[189])MOV(6,Inprocess_Index)OTL(Port_Data.Port_Write.[Port])OTL(Local_Control.11);
   89: NOP();
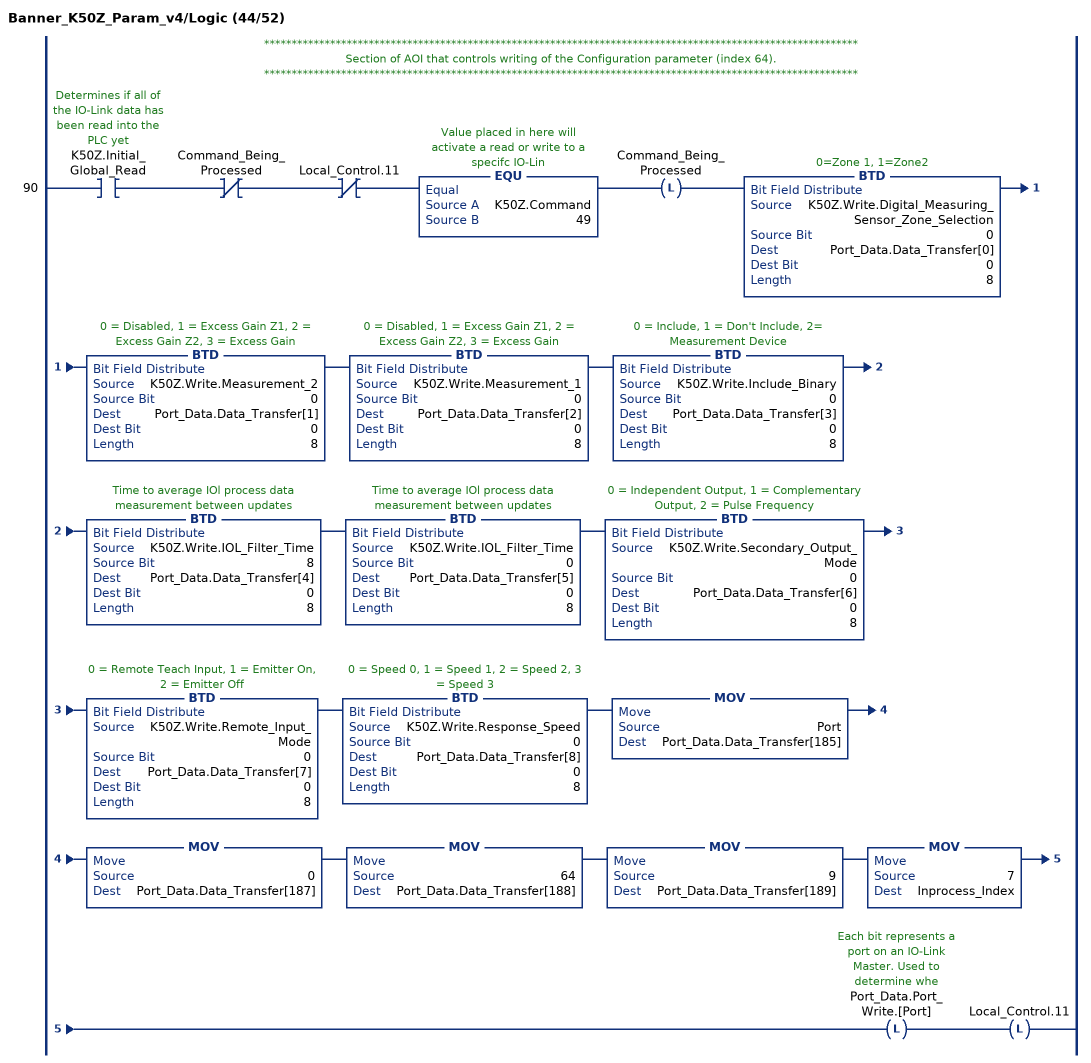
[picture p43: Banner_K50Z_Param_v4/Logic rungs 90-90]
   // ************************************************************************************************************
   // Section of AOI that controls writing of the Configuration parameter (index 64).
   // ************************************************************************************************************
   90: XIC(K50Z.Initial_Global_Read)XIO(Command_Being_Processed)XIO(Local_Control.11)EQU(K50Z.Command,49)OTL(Command_Being_Processed)BTD(K50Z.Write.Digital_Measuring_Sensor_Zone_Selection,0,Port_Data.Data_Transfer[0],0,8)BTD(K50Z.Write.Measurement_2,0,Port_Data.Data_Transfer[1],0,8)BTD(K50Z.Write.Measurement_1,0,Port_Data.Data_Transfer[2],0,8)BTD(K50Z.Write.Include_Binary,0,Port_Data.Data_Transfer[3],0,8)BTD(K50Z.Write.IOL_Filter_Time,8,Port_Data.Data_Transfer[4],0,8)BTD(K50Z.Write.IOL_Filter_Time,0,Port_Data.Data_Transfer[5],0,8)BTD(K50Z.Write.Secondary_Output_Mode,0,Port_Data.Data_Transfer[6],0,8)BTD(K50Z.Write.Remote_Input_Mode,0,Port_Data.Data_Transfer[7],0,8)BTD(K50Z.Write.Response_Speed,0,Port_Data.Data_Transfer[8],0,8)MOV(Port,Port_Data.Data_Transfer[185])MOV(0,Port_Data.Data_Transfer[187])MOV(64,Port_Data.Data_Transfer[188])MOV(9,Port_Data.Data_Transfer[189])MOV(7,Inprocess_Index)OTL(Port_Data.Port_Write.[Port])OTL(Local_Control.11);
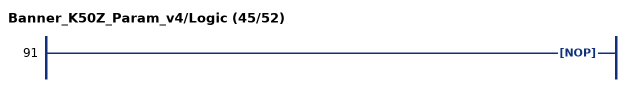
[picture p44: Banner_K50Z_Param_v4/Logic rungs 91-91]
   91: NOP();
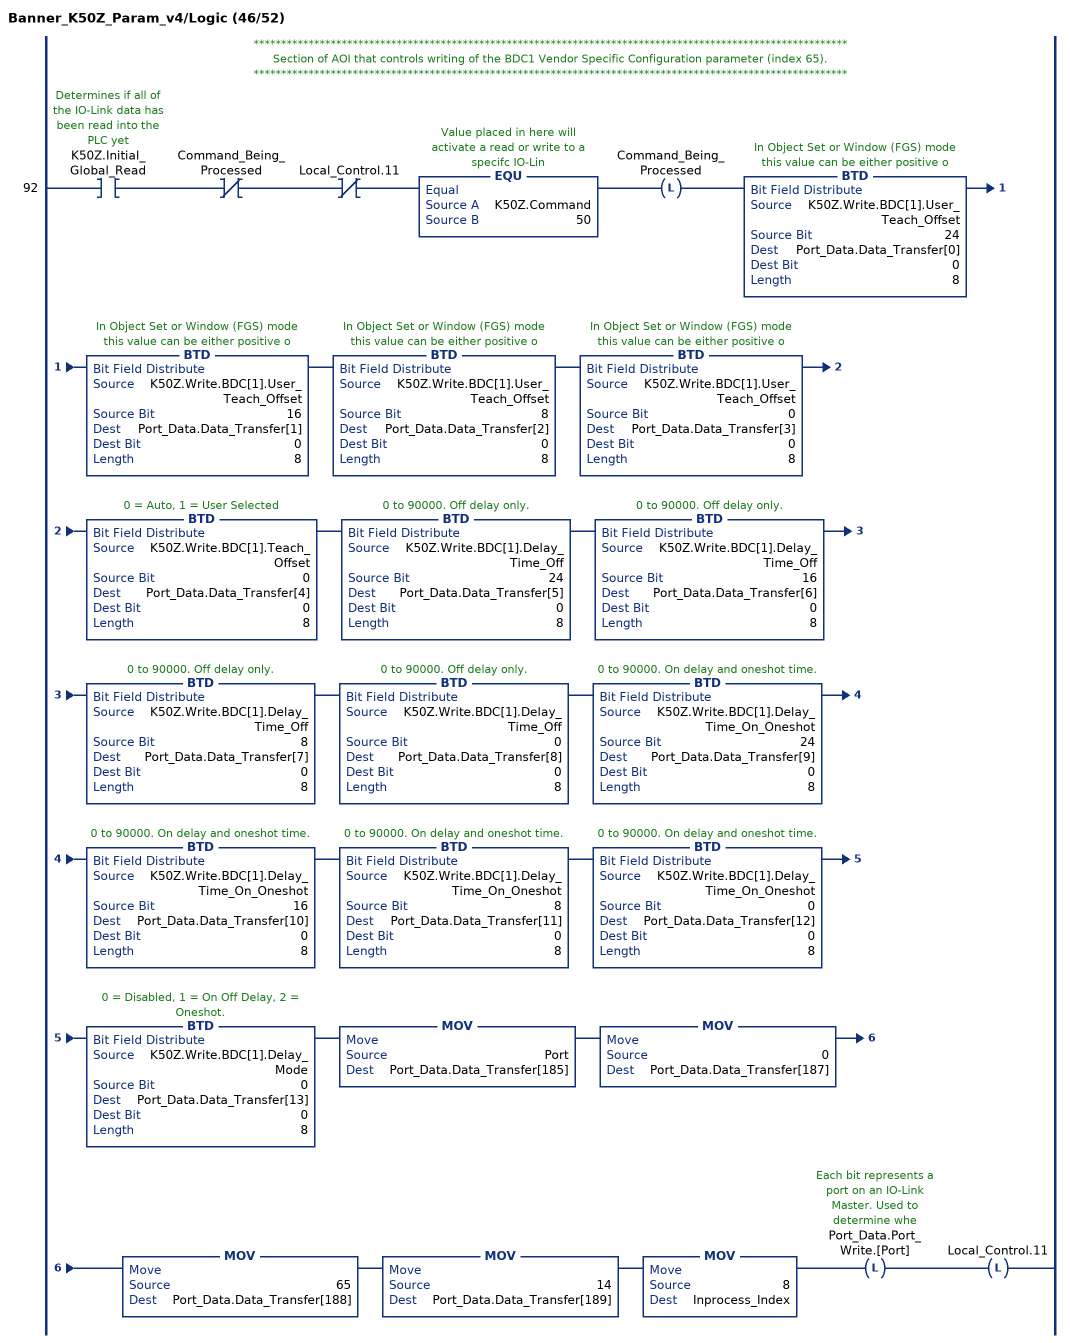
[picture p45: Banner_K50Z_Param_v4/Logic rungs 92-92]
   // ************************************************************************************************************
   // Section of AOI that controls writing of the BDC1 Vendor Specific Configuration parameter (index 65).
   // ************************************************************************************************************
   92: XIC(K50Z.Initial_Global_Read)XIO(Command_Being_Processed)XIO(Local_Control.11)EQU(K50Z.Command,50)OTL(Command_Being_Processed)BTD(K50Z.Write.BDC[1].User_Teach_Offset,24,Port_Data.Data_Transfer[0],0,8)BTD(K50Z.Write.BDC[1].User_Teach_Offset,16,Port_Data.Data_Transfer[1],0,8)BTD(K50Z.Write.BDC[1].User_Teach_Offset,8,Port_Data.Data_Transfer[2],0,8)BTD(K50Z.Write.BDC[1].User_Teach_Offset,0,Port_Data.Data_Transfer[3],0,8)BTD(K50Z.Write.BDC[1].Teach_Offset,0,Port_Data.Data_Transfer[4],0,8)BTD(K50Z.Write.BDC[1].Delay_Time_Off,24,Port_Data.Data_Transfer[5],0,8)BTD(K50Z.Write.BDC[1].Delay_Time_Off,16,Port_Data.Data_Transfer[6],0,8)BTD(K50Z.Write.BDC[1].Delay_Time_Off,8,Port_Data.Data_Transfer[7],0,8)BTD(K50Z.Write.BDC[1].Delay_Time_Off,0,Port_Data.Data_Transfer[8],0,8)BTD(K50Z.Write.BDC[1].Delay_Time_On_Oneshot,24,Port_Data.Data_Transfer[9],0,8)BTD(K50Z.Write.BDC[1].Delay_Time_On_Oneshot,16,Port_Data.Data_Transfer[10],0,8)BTD(K50Z.Write.BDC[1].Delay_Time_On_Oneshot,8,Port_Data.Data_Transfer[11],0,8)BTD(K50Z.Write.BDC[1].Delay_Time_On_Oneshot,0,Port_Data.Data_Transfer[12],0,8)BTD(K50Z.Write.BDC[1].Delay_Mode,0,Port_Data.Data_Transfer[13],0,8)MOV(Port,Port_Data.Data_Transfer[185])MOV(0,Port_Data.Data_Transfer[187])MOV(65,Port_Data.Data_Transfer[188])MOV(14,Port_Data.Data_Transfer[189])MOV(8,Inprocess_Index)OTL(Port_Data.Port_Write.[Port])OTL(Local_Control.11);
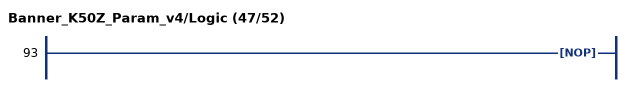
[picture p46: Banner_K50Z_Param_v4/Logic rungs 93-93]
   93: NOP();
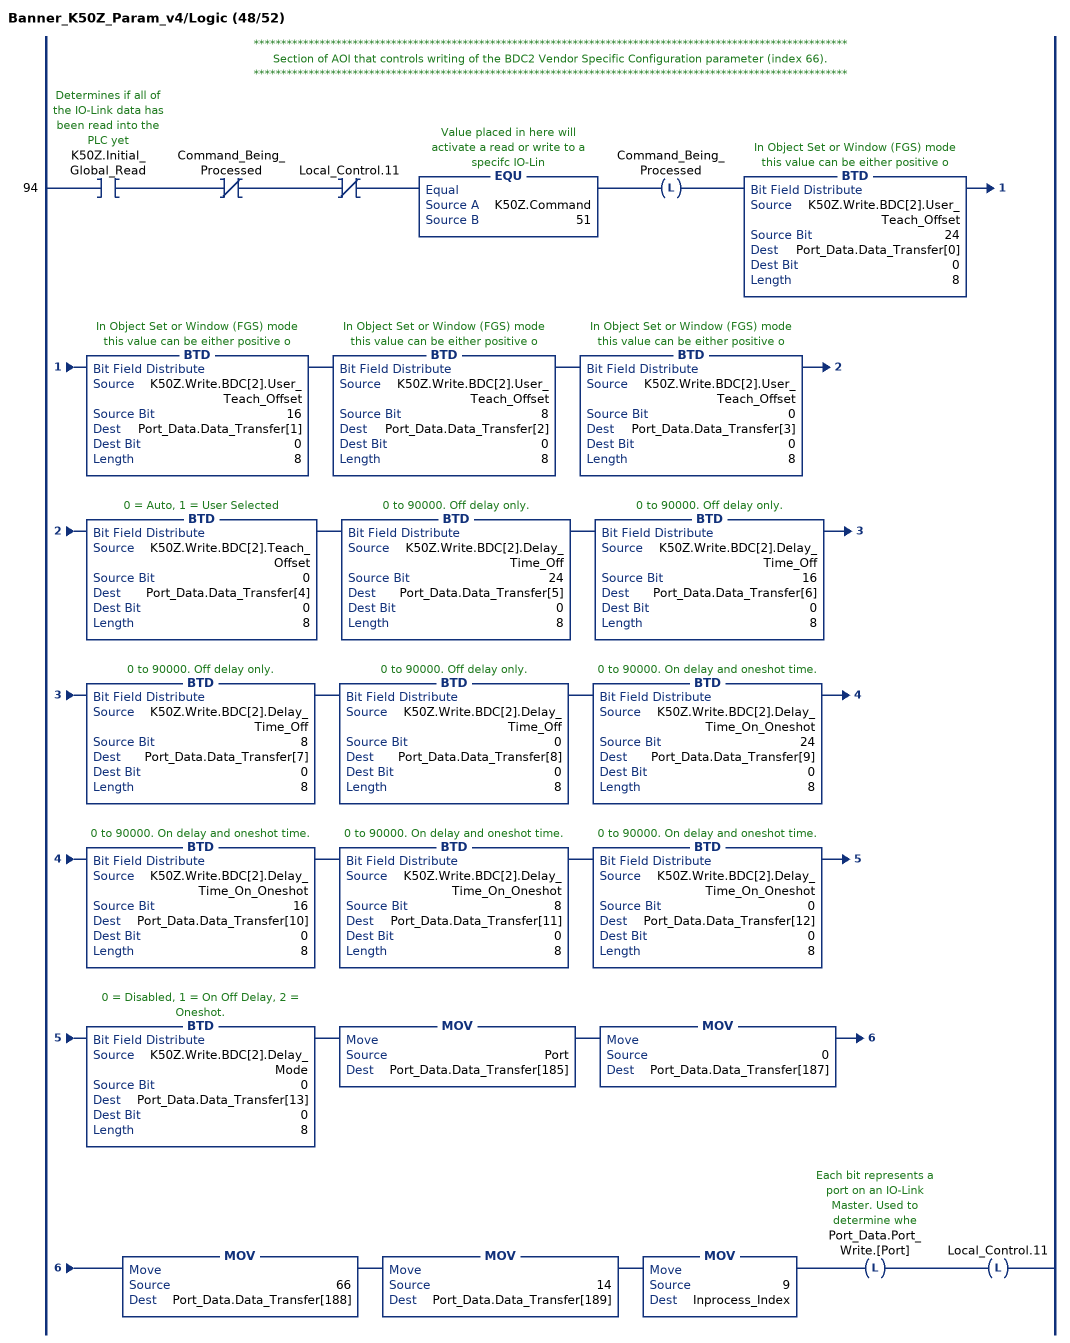
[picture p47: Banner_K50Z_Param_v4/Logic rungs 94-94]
   // ************************************************************************************************************
   // Section of AOI that controls writing of the BDC2 Vendor Specific Configuration parameter (index 66).
   // ************************************************************************************************************
   94: XIC(K50Z.Initial_Global_Read)XIO(Command_Being_Processed)XIO(Local_Control.11)EQU(K50Z.Command,51)OTL(Command_Being_Processed)BTD(K50Z.Write.BDC[2].User_Teach_Offset,24,Port_Data.Data_Transfer[0],0,8)BTD(K50Z.Write.BDC[2].User_Teach_Offset,16,Port_Data.Data_Transfer[1],0,8)BTD(K50Z.Write.BDC[2].User_Teach_Offset,8,Port_Data.Data_Transfer[2],0,8)BTD(K50Z.Write.BDC[2].User_Teach_Offset,0,Port_Data.Data_Transfer[3],0,8)BTD(K50Z.Write.BDC[2].Teach_Offset,0,Port_Data.Data_Transfer[4],0,8)BTD(K50Z.Write.BDC[2].Delay_Time_Off,24,Port_Data.Data_Transfer[5],0,8)BTD(K50Z.Write.BDC[2].Delay_Time_Off,16,Port_Data.Data_Transfer[6],0,8)BTD(K50Z.Write.BDC[2].Delay_Time_Off,8,Port_Data.Data_Transfer[7],0,8)BTD(K50Z.Write.BDC[2].Delay_Time_Off,0,Port_Data.Data_Transfer[8],0,8)BTD(K50Z.Write.BDC[2].Delay_Time_On_Oneshot,24,Port_Data.Data_Transfer[9],0,8)BTD(K50Z.Write.BDC[2].Delay_Time_On_Oneshot,16,Port_Data.Data_Transfer[10],0,8)BTD(K50Z.Write.BDC[2].Delay_Time_On_Oneshot,8,Port_Data.Data_Transfer[11],0,8)BTD(K50Z.Write.BDC[2].Delay_Time_On_Oneshot,0,Port_Data.Data_Transfer[12],0,8)BTD(K50Z.Write.BDC[2].Delay_Mode,0,Port_Data.Data_Transfer[13],0,8)MOV(Port,Port_Data.Data_Transfer[185])MOV(0,Port_Data.Data_Transfer[187])MOV(66,Port_Data.Data_Transfer[188])MOV(14,Port_Data.Data_Transfer[189])MOV(9,Inprocess_Index)OTL(Port_Data.Port_Write.[Port])OTL(Local_Control.11);
